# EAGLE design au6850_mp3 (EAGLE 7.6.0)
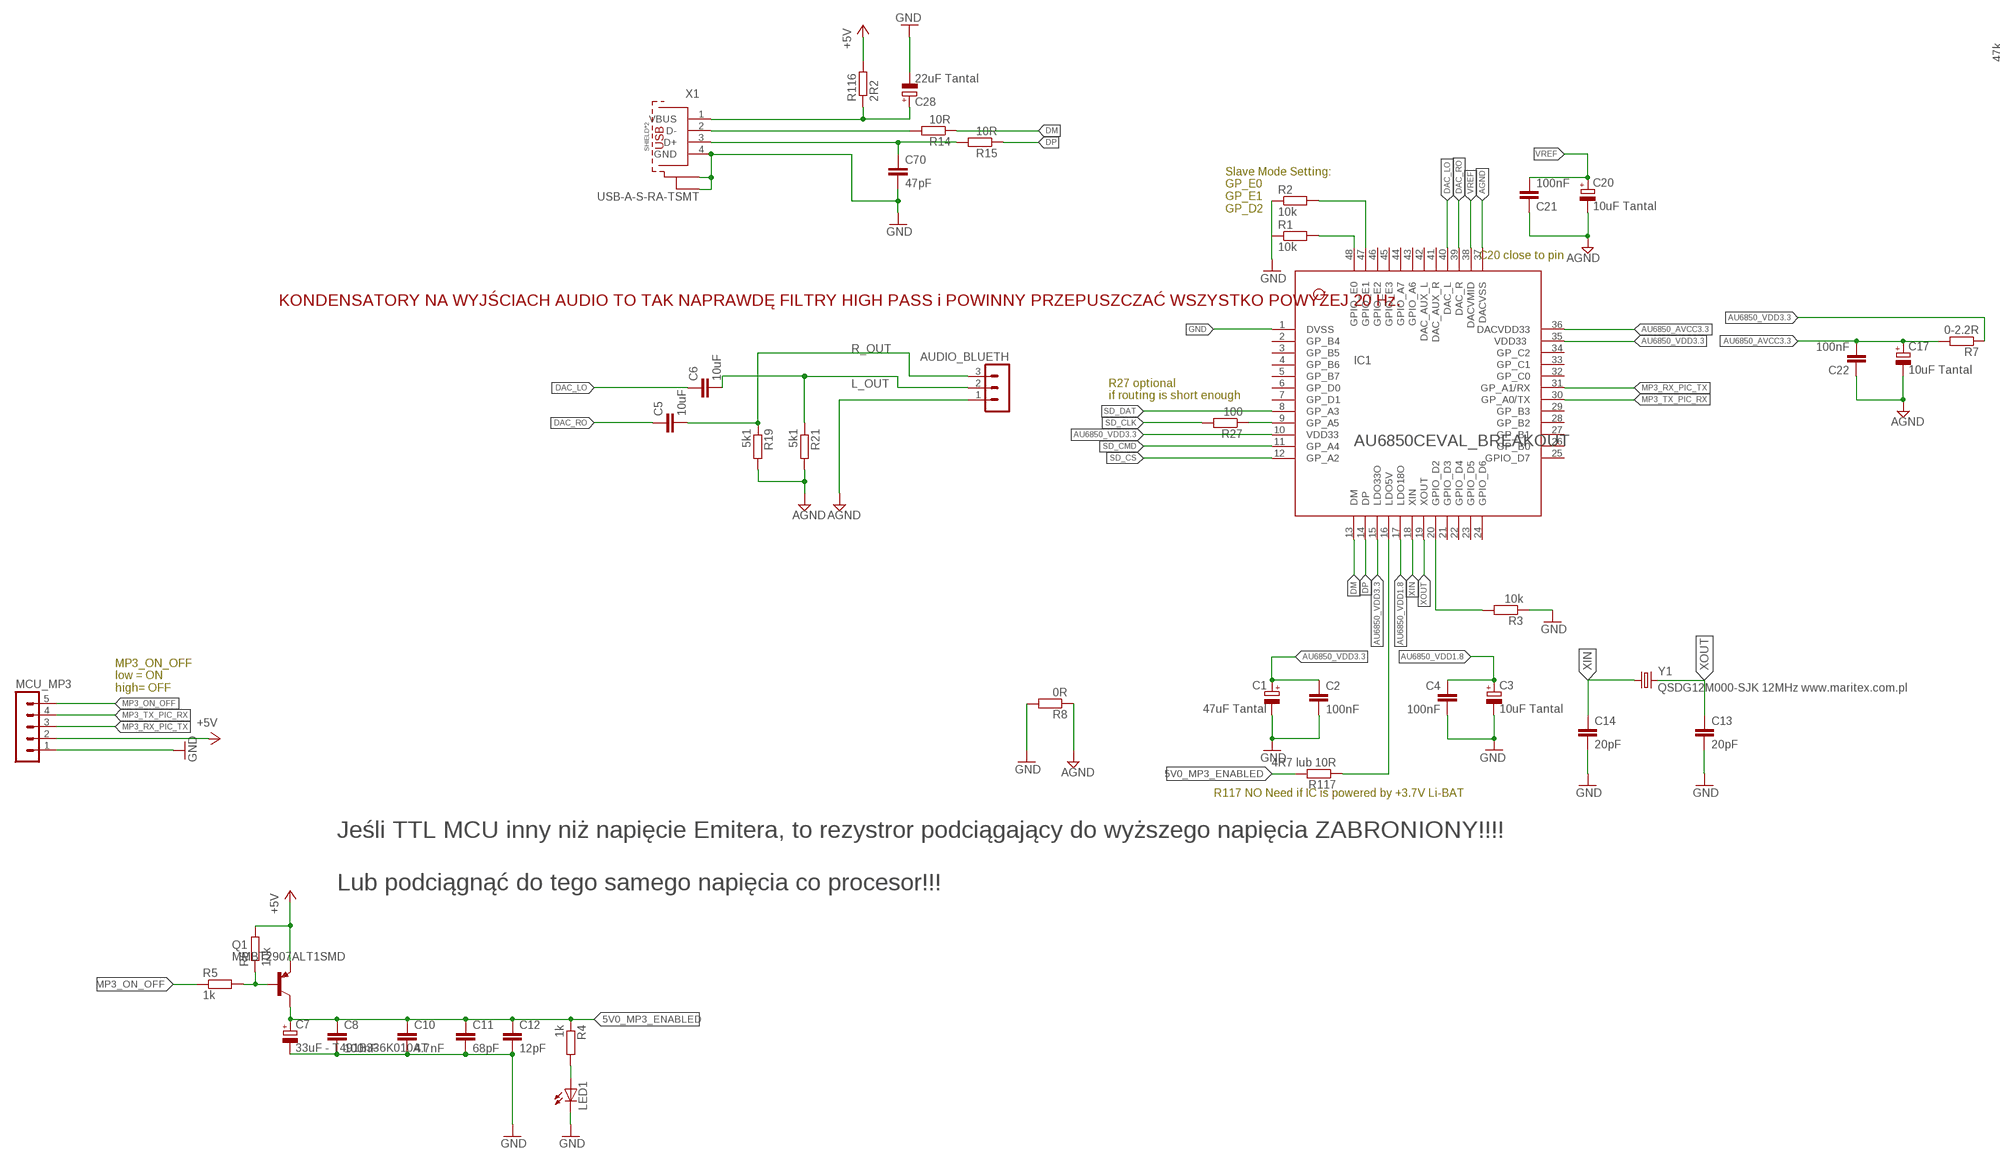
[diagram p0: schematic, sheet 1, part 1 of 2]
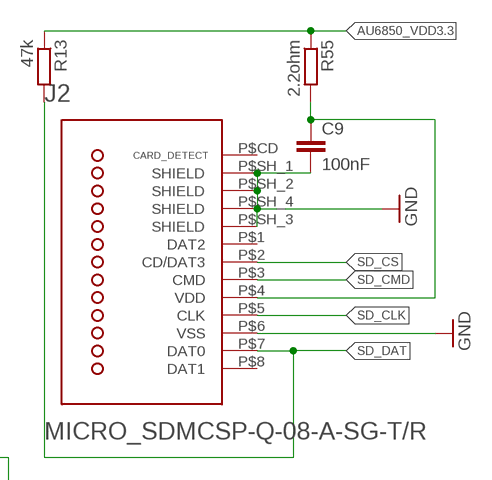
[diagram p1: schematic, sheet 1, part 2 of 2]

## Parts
AUDIO_BLUETH  MA03-1  [MA03-1]
C1  47uF Tantal  CPOL-EUB/3528-21R  [B/3528-21R]
C2  100nF  C-EUC0805  [C0805]
C3  10uF Tantal  CPOL-EUB/3528-21R  [B/3528-21R]
C4  100nF  C-EUC0805  [C0805]
C5  10uF  C-EUC0805  [C0805]
C6  10uF  C-EUC0805  [C0805]
C7  33uF - T491B336K010AT  CPOL-EUSMCB  [SMC_B]
C8  100nF  C-EUC0805  [C0805]
C9  100nF  C-EUC0805  [C0805]
C10  4.7nF  C-EUC0805  [C0805]
C11  68pF  C-EUC0805  [C0805]
C12  12pF  C-EUC0603K  [C0603K]
C13  20pF  C-EUC0805  [C0805]
C14  20pF  C-EUC0805  [C0805]
C17  10uF Tantal  CPOL-EUB/3528-21R  [B/3528-21R]
C20  10uF Tantal  CPOL-EUB/3528-21R  [B/3528-21R]
C21  100nF  C-EUC0805  [C0805]
C22  100nF  C-EUC0805  [C0805]
C28  22uF Tantal  CPOL-EUSMCB  [SMC_B]
C70  47pF  C-EUC0805  [C0805]
IC1  AU6850CEVAL_BREAKOUT  [LQFP48-7BREAKOUT]
J2  MICRO_SDMCSP-Q-08-A-SG-T/R  [MICRO_SD_8PINS]
LED1  LED3MM  [LED3MM]
MCU_MP3  MA05-1  [MA05-1]
Q1  MMBT2907ALT1SMD  [SOT23-BEC]
R1  10k  R-EU_R0805  [R0805]
R2  10k  R-EU_R0805  [R0805]
R3  10k  R-EU_R0805  [R0805]
R4  1k  R-EU_M0805  [M0805]
R5  1k  R-EU_M0805  [M0805]
R6  10k  R-EU_M0805  [M0805]
R7  0-2.2R  R-EU_R0805  [R0805]
R8  0R  R-EU_R0805  [R0805]
R13  47k  R-EU_R0805  [R0805]
R14  10R  R-EU_R0805  [R0805]
R15  10R  R-EU_R0805  [R0805]
R19  5k1  R-EU_R0805  [R0805]
R21  5k1  R-EU_R0805  [R0805]
R27  100  R-EU_R0805  [R0805]
R55  2.2ohm  R-EU_R0805  [R0805]
R116  2R2  R-EU_R0805  [R0805]
R117  4R7 lub 10R  R-EU_R0805  [R0805]
X1  USB-A-S-RA-TSMT  [USB-A-S-RA-TSMT]
Y1  QSDG12M000-SJK 12MHz www.maritex.com.pl  CRYSTALSMD  [HC49UP]

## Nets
5V0_MP3_ENABLED: C7.+ C8.1 C10.1 C11.1 C12.1 Q1.C R4.1 R117.2
+5V: MCU_MP3.2 Q1.E R6.2 R116.2
AGND: AUDIO_BLUETH.1 C17.- C20.- C21.1 C22.1 IC1.37(DACVSS) R8.1 R19.2 R21.2
AU6850_AVCC3.3: C17.+ C22.2 IC1.36(DACVDD33) R7.2
AU6850_VDD1.8: C3.+ C4.1 IC1.17(LDO18O)
AU6850_VDD3.3: C1.+ C2.1 IC1.10(VDD33) IC1.15(LDO33O) IC1.35(VDD33) R7.1 R13.1 R55.1
DAC_LO: C6.1 IC1.40(DAC_L)
DAC_RO: C5.1 IC1.39(DAC_R)
DM: IC1.13(DM) R14.1
DP: IC1.14(DP) R15.1
GND: C1.- C2.2 C3.- C4.2 C7.- C8.2 C9.2 C10.2 C11.2 C12.2 C13.2 C14.2 C28.- C70.2 IC1.1(DVSS) J2.P$6(VSS) J2.P$SH_1(1_GND_PAD) J2.P$SH_2(2_GND_PAD) J2.P$SH_3(3_GND_PAD) J2.P$SH_4(4_GND_PAD) LED1.K(C) MCU_MP3.1 R1.1 R2.1 R3.1 R8.2 X1.4(GND) X1.5(SH1) X1.6(SH2)
L_OUT: AUDIO_BLUETH.2 C6.2 R21.1
MP3_ON_OFF: MCU_MP3.5 R5.1
MP3_RX_PIC_TX: IC1.31(GP_A1/RX) MCU_MP3.3
MP3_TX_PIC_RX: IC1.30(GP_A0/TX) MCU_MP3.4
N$1: LED1.A R4.2
N$2: Q1.B R5.2 R6.1
N$4: IC1.16(LDO5V) R117.1
N$5: IC1.9(GP_A5) R27.1
N$8: C28.+ R116.1 X1.1(VBUS)
N$9: C70.1 R15.2 X1.3(D+)
N$10: R14.2 X1.2(D-)
N$14: C9.1 J2.P$4(VDD) R55.2
R_OUT: AUDIO_BLUETH.3 C5.2 R19.1
SD_CLK: J2.P$5(CLK) R27.2
SD_CMD: IC1.11(GP_A4) J2.P$3(CMD)
SD_CS: IC1.12(GP_A2) J2.P$2(CD/DAT3)
SD_DAT: IC1.8(GP_A3) J2.P$7(DAT0) R13.2
SLAVE_D2: IC1.20(GPIO_D2) R3.2
SLAVE_E0: IC1.48(GPIO_E0) R1.2
SLAVE_E1: IC1.47(GPIO_E1) R2.2
VREF: C20.+ C21.2 IC1.38(DACVMID)
XIN: C14.1 IC1.18(XIN) Y1.1
XOUT: C13.1 IC1.19(XOUT) Y1.2
Unconnected: IC1.2(GP_B4) IC1.3(GP_B5) IC1.4(GP_B6) IC1.5(GP_B7) IC1.6(GP_D0) IC1.7(GP_D1) IC1.21(GPIO_D3) IC1.22(GPIO_D4) IC1.23(GPIO_D5) IC1.24(GPIO_D6) IC1.25(GPIO_D7) IC1.26(GP_B0) IC1.27(GP_B1) IC1.28(GP_B2) IC1.29(GP_B3) IC1.32(GP_C0) IC1.33(GP_C1) IC1.34(GP_C2) IC1.41(DAC_AUX_R) IC1.42(DAC_AUX_L) IC1.43(GPIO_A6) IC1.44(GPIO_A7) IC1.45(GPIO_E3) IC1.46(GPIO_E2) J2.P$1(DAT2) J2.P$8(DAT1) J2.P$CD(CARD_DETECT_SW)

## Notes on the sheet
- Slave Mode Setting:
  GP_E0
  GP_E1
  GP_D2
- C20 close to pin
- KONDENSATORY NA WYJŚCIACH AUDIO TO TAK NAPRAWDĘ FILTRY HIGH PASS i POWINNY PRZEPUSZCZAĆ WSZYSTKO POWYŻEJ 20 Hz.
- R27 optional
  if routing is short enough
- MP3_ON_OFF
  low = ON
  high= OFF
- R117 NO Need if IC is powered by +3.7V Li-BAT
- Jeśli TTL MCU inny niż napięcie Emitera, to rezystror podciągający do wyższego napięcia ZABRONIONY!!!!
  
  Lub podciągnąć do tego samego napięcia co procesor!!!

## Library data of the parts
AUDIO_BLUETH = con-lstb:MA03-1: PIN HEADER; OC_FARNELL: unknown; OC_NEWARK: unknown
C1 = rcl:CPOL-EU: POLARIZED CAPACITOR, European symbol; PARTNUM: TAJB476K010R; SUPPLIER: TME
C2 C4-C6 C21 C22 = rcl:C-EU: CAPACITOR, European symbol
C3 = rcl:CPOL-EU: POLARIZED CAPACITOR, European symbol; PARTNUM: TAJA106K010R; SUPPLIER: TME
C7 = resistor:CPOL-EU: POLARIZED CAPACITOR, European symbol; PARTNUM: TAJB336K010R; SUPPLIER: TME
C8-C14 C70 = resistor:C-EU: CAPACITOR, European symbol
C17 C20 = rcl:CPOL-EU: POLARIZED CAPACITOR, European symbol
C28 = rcl:CPOL-EU: POLARIZED CAPACITOR, European symbol; PARTNUM: TAJB226M010R; SUPPLIER: TME
IC1 = mvsilicon:AU6850C
J2 = ADAM_TECH_SD_Card:MICRO_SD: Adam Tech; PARTNUM: MCSP-Q-08-A-SG-T/R; SUPPLIER: TME
LED1 = led:LED: LED
MCU_MP3 = con-lstb:MA05-1: PIN HEADER; OC_FARNELL: unknown; OC_NEWARK: unknown
Q1 = transistor-pnp:MMBT2907*: PNP Transistror
R1-R8 R13-R15 R19 R21 R27 R55 R116 R117 = rcl:R-EU_: RESISTOR, European symbol
X1 = ADAM_TECH_USB-A-S-RA-TSMT:USB-A-S-RA-TSMT: MULTICOMP - USB-A-S-RA-TSMT - USB, 3.0 TYPE A, RECEPTACLE, SMT CUI -UJ2-AH-1-SMT-TR, 3.0 TYPE A, RECEPTACLE, SMT AdamTech - USB-A-S-RA-TSMT - USB, 3.0 TYPE A, RECEPTACLE, SMT Source: Datasheet; DESCRIPTION: MULTICOMP - USB-A-S-RA-TSMT - USB, 3.0 TYPE A, RECEPTACLE, SMT; HEIGHT: mm; MANUFACTURER_NAME: MULTICOMP; MANUFACTURER_PART_NUMBER: USB-A-S-RA-TSMT
Y1 = SparkFun-FreqCtrl:CRYSTAL: Various standard crystals. Proven footprints. Spark Fun Electronics SKU : COM-00534; PARTNUM: 12.00M-SMDHC49S; SUPPLIER: TME

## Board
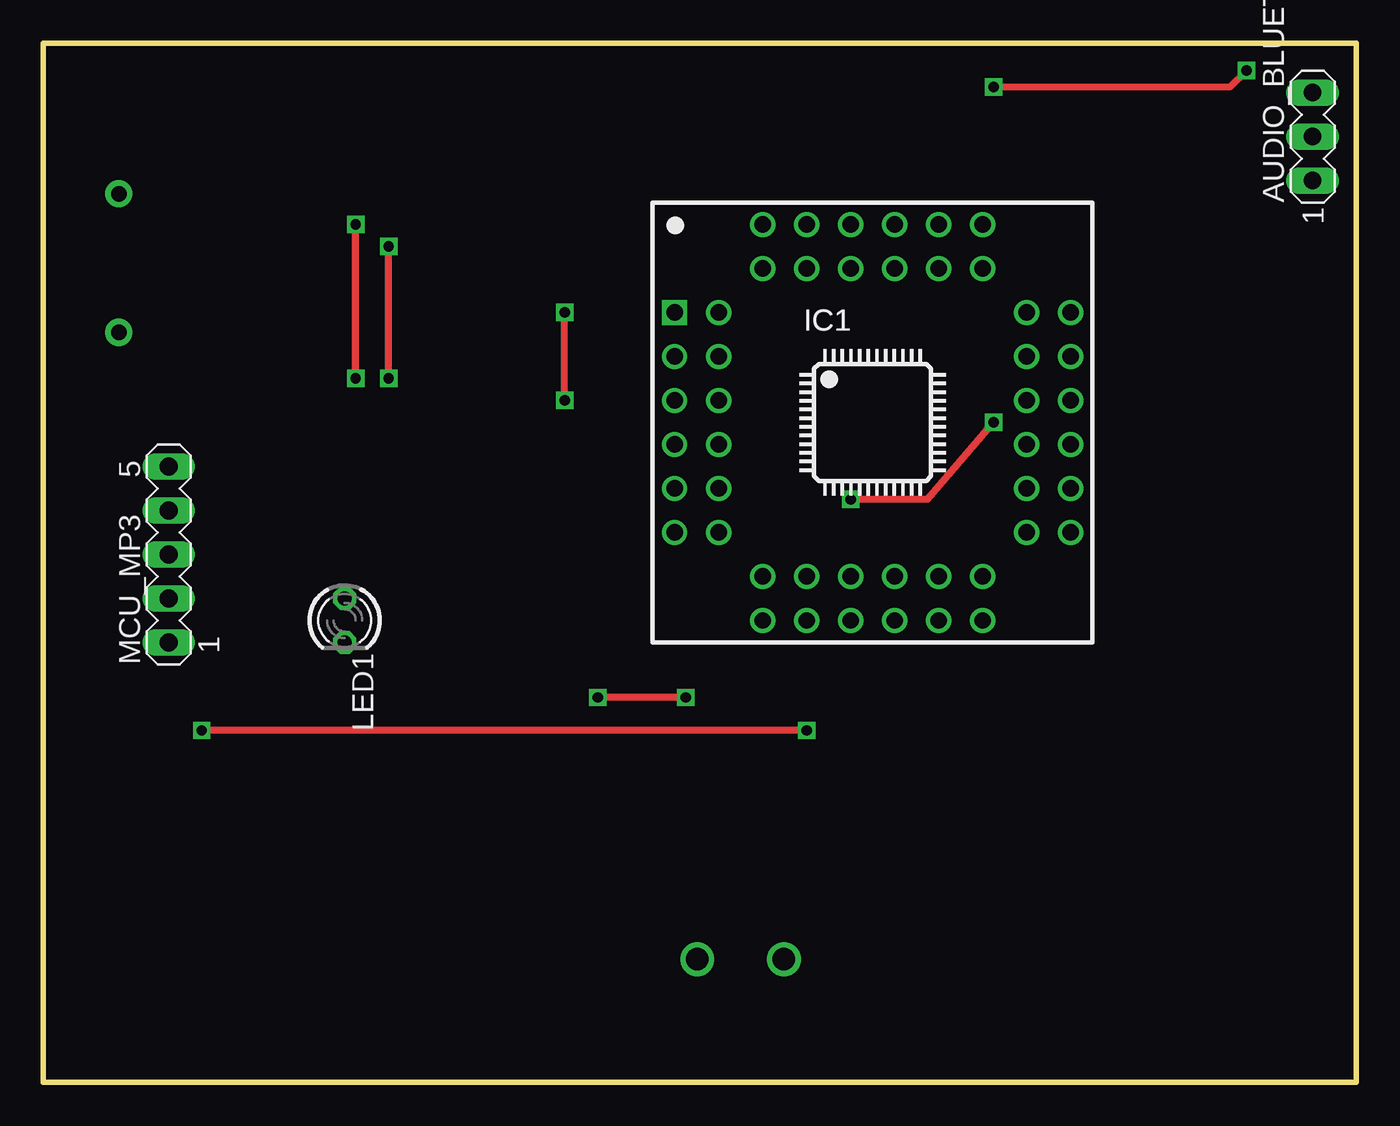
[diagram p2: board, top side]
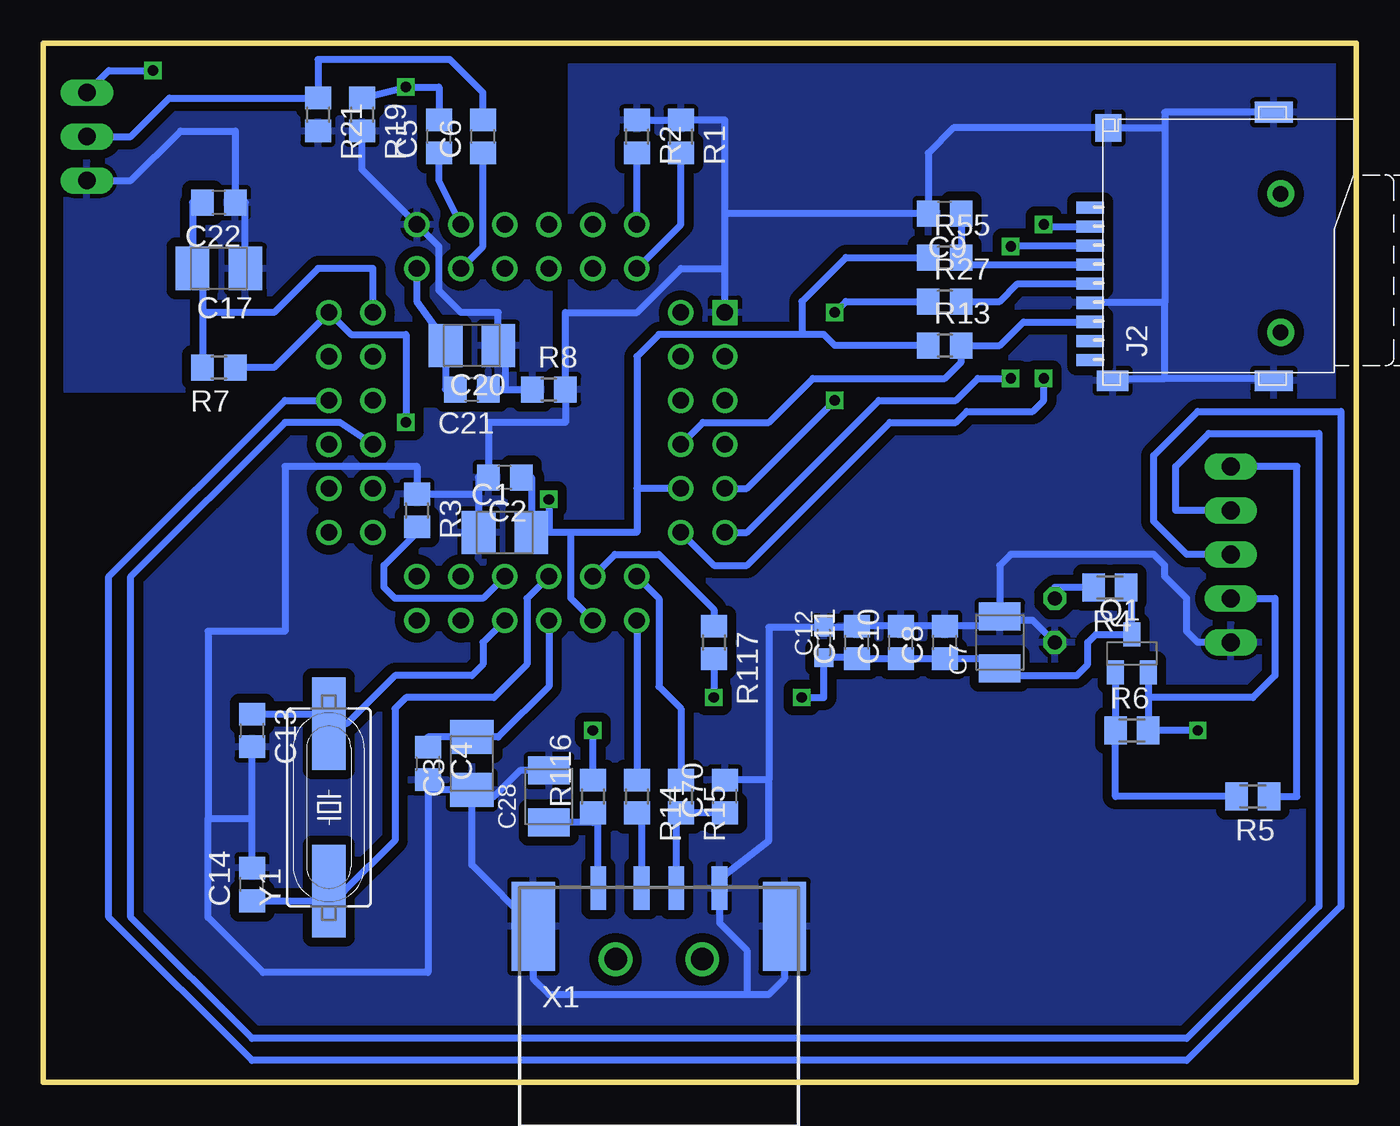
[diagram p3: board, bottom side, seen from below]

Size 75.8 x 59.99 mm. Coordinates in mm from the lower left corner, seen from the top.
Outline: 0,0 75.8,0 75.8,59.99 0,59.99 0,0
Copper layers (1*16): Top 0.035mm / dielectric 1.5mm / Bottom 0.035mm
Design rules "default": minimum track width 10mil, minimum drill 24mil, track to track 8mil, track to pad 8mil, pad to pad 8mil, via to via 8mil, smd to smd 8mil, copper to edge 40mil, drill to drill 8mil, minimum pad ring 10mil, minimum via ring 8mil, stop-mask expansion 4mil, vias tented up to drill 0mil, thermal gap 10mil

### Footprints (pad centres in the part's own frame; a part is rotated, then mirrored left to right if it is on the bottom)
MA03-1 = drill 1.016 long: 1 -2.54,0; 2 0,0; 3 2.54,0
B/3528-21R = smd 1.95 x 2.5: + 1.525,0; - -1.525,0
C0805 = smd 1.3 x 1.5: 1 -0.95,0; 2 0.95,0
SMC_B = smd 1.6 x 2.4: + -1.5,0; - 1.5,0
C0603K = smd 1.05 x 1.08: 1 -0.875,0; 2 0.875,0
LQFP48-7BREAKOUT = drill 0.95 square: 1 -11.43,6.35 | drill 0.95: 2 -8.89,6.35; 3 -11.43,3.81; 4 -8.89,3.81; 5 -11.43,1.27; 6 -8.89,1.27; 7 -11.43,-1.27; 8 -8.89,-1.27; 9 -11.43,-3.81; 10 -8.89,-3.81; 11 -11.43,-6.35; 12 -8.89,-6.35; 13 -6.35,-11.43; 14 -6.35,-8.89; 15 -3.81,-11.43; 16 -3.81,-8.89; 17 -1.27,-11.43; 18 -1.27,-8.89; 19 1.27,-11.43; 20 1.27,-8.89; 21 3.81,-11.43; 22 3.81,-8.89; 23 6.35,-11.43; 24 6.35,-8.89; 25 11.43,-6.35; 26 8.89,-6.35; 27 11.43,-3.81; 28 8.89,-3.81; 29 11.43,-1.27; 30 8.89,-1.27; 31 11.43,1.27; 32 8.89,1.27; 33 11.43,3.81; 34 8.89,3.81; 35 11.43,6.35; 36 8.89,6.35; 37 6.35,11.43; 38 6.35,8.89; 39 3.81,11.43; 40 3.81,8.89; 41 1.27,11.43; 42 1.27,8.89; 43 -1.27,11.43; 44 -1.27,8.89; 45 -3.81,11.43; 46 -3.81,8.89; 47 -6.35,11.43; 48 -6.35,8.89
MICRO_SD_8PINS = drill 0.9 pad 1.575: 1 -4.95,-10.5; 15 3.05,-10.5 | smd 0.7 x 1.6: P$1 2.25,0.5; P$2 1.15,0.5; P$3 0.05,0.5; P$4 -1.05,0.5; P$5 -2.15,0.5; P$6 -3.25,0.5; P$7 -4.35,0.5; P$8 -5.45,0.5; P$CD -6.55,0.5 | smd 1.2 x 2.2: P$SH_1 -7.75,-10.1; P$SH_2 7.75,-10.1 | smd 1.2 x 1.8: P$SH_3 -7.75,-0.8 | smd 1.6 x 1.5: P$SH_4 6.85,-0.55
LED3MM = drill 0.813 octagon: A -1.27,0; K 1.27,0
MA05-1 = drill 1.016 long: 1 -5.08,0; 2 -2.54,0; 3 0,0; 4 2.54,0; 5 5.08,0
SOT23-BEC = smd 1 x 1.4: B -0.95,-1.1; C 0,1.1; E 0.95,-1.1
R0805 = smd 1.3 x 1.5: 1 -0.95,0; 2 0.95,0
M0805 = smd 1.3 x 1.6: 1 -0.95,0; 2 0.95,0
USB-A-S-RA-TSMT = smd 0.9 x 2.5: 1 -3.5,13.75; 2 -1,13.75; 3 1,13.75; 4 3.5,13.75 | smd 2.5 x 5.15: 5 -7.25,11.55; 6 7.25,11.55 | drill 1.3 pad 1.95: 7 -2.5,9.65; 8 2.5,9.65
HC49UP = smd 5.334 x 1.93: 1 -4.826,0; 2 4.826,0

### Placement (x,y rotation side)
AUDIO_BLUETH  73.28,54.61 90 top
C1  49.15,31.75 0 bottom
C2  49.15,34.93 180 bottom
C3  51.05,18.41 90 bottom
C4  53.59,18.41 270 bottom
C5  52.96,54.61 90 bottom
C6  50.42,54.61 90 bottom
C7  20.57,25.4 90 bottom
C8  23.75,25.4 90 bottom
C9  23.75,50.16 180 bottom
C10  26.29,25.4 90 bottom
C11  28.83,25.4 90 bottom
C12  30.73,25.4 90 bottom
C13  63.75,20.32 270 bottom
C14  63.75,11.43 90 bottom
C17  65.66,46.99 180 bottom
C20  51.05,42.55 180 bottom
C21  51.05,40.01 180 bottom
C22  65.66,50.8 180 bottom
C28  46.61,16.51 90 bottom
C70  36.45,16.51 90 bottom
IC1  47.88,38.1 0 top
J2  14.86,48.26 90 bottom
LED1  17.4,26.67 270 top
MCU_MP3  7.24,30.48 90 top
Q1  12.95,24.77 0 bottom
R1  38.99,54.61 270 bottom
R2  41.53,54.61 270 bottom
R3  54.23,33.02 270 bottom
R4  14.22,28.57 180 bottom
R5  5.97,16.51 180 bottom
R6  12.95,20.32 0 bottom
R7  65.66,41.27 180 bottom
R8  46.61,40.01 0 bottom
R13  23.75,42.55 0 bottom
R14  41.53,16.51 270 bottom
R15  38.99,16.51 270 bottom
R19  57.4,55.88 270 bottom
R21  59.94,55.88 270 bottom
R27  23.75,45.09 0 bottom
R55  23.75,47.62 0 bottom
R116  44.07,16.51 90 bottom
R117  37.08,25.4 270 bottom
X1  40.26,-2.54 0 bottom
Y1  59.31,15.88 90 bottom

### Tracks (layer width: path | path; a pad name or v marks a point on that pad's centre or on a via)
5V0_MP3_ENABLED  (via drill 0.6)
  Top 0.406: v37.08,22.23 v32,22.23
  Bottom 0.406: R4.1 arc90 12.95,28.26 Q1.C 15.03,25.87 15.49,25.4 15.49,24.13 16.13,23.5 20.17,23.5 C7.+ 21.12,24.45 C8.1 C10.1 C11.1 28.9,24.53 C12.1 30.73,22.23 v32,22.23 | R117.2 v37.08,22.23
+5V  (via drill 0.6)
  Top 0.406: v44.07,20.32 v9.14,20.32
  Bottom 0.406: Q1.E 12,22.23 | 12,22.23 R6.2 v9.14,20.32 | MCU_MP3.2 4.7,27.94 4.7,23.5 5.97,22.23 12,22.23 | R116.2 v44.07,20.32
AGND
  Bottom 0.406: AUDIO_BLUETH.1 70.74,52.07 67.88,54.93 64.71,54.93 C22.1 | C22.1 64.39,50.8 | C17.- 64.13,50.8 C22.1 | C21.1 49.15,40.01 | 49.15,40.01 R8.1 | 49.15,40.01 49.15,42.16 C20.- 49.53,44.45 51.69,44.45 52.96,45.72 52.96,48.26 IC1.37 57.4,52.7 R19.2
  pour Bottom (isolate 0.533): 46.61,40.01 79.63,40.01 79.63,62.23 46.61,62.23
AU6850_AVCC3.3
  Bottom 0.406: C22.2 67.18,50.8 C17.+ 66.61,46.99 66.61,44.45 | 66.61,44.45 R7.2 | IC1.36 56.77,46.99 59.94,46.99 62.48,44.45 66.61,44.45
AU6850_VDD1.8
  Bottom 0.406: IC1.17 46.61,22.86 49.53,19.94 C3.+ 53.59,19.94 C4.1
AU6850_VDD3.3  (via drill 0.6)
  Top 0.406: v54.86,38.1 51.05,33.66 v46.61,33.66
  Bottom 0.406: IC1.15 45.34,27.94 45.34,31.75 | IC1.10 41.53,34.29 | R7.1 62.48,41.27 IC1.35 58.04,43.18 54.86,43.18 v54.86,38.1 | R13.1 30.1,42.55 30.73,43.18 32,43.18 | 32,43.18 40.26,43.18 41.53,41.91 41.53,34.29 | 32,43.18 32,45.09 29.46,47.62 R55.1 | 41.53,34.29 41.53,31.75 45.34,31.75 | 45.34,31.75 46.61,31.75 | 46.61,31.75 C1.+ 47.62,34.93 C2.1 | v46.61,33.66 46.61,31.75
DAC_LO
  Bottom 0.406: IC1.40 50.42,48.26 C6.1
DAC_RO
  Bottom 0.406: IC1.39 52.96,52.07 C5.1
DM
  Bottom 0.406: IC1.13 R14.1
DP
  Bottom 0.406: IC1.14 40.26,27.94 40.26,22.86 38.99,21.59 R15.1
GND
  Bottom 0.406: R2.1 R1.1 36.45,55.56 36.45,50.16 | C28.- 48.28,18.01 49.78,16.51 50.67,16.51 C3.- | 35.18,5.08 46.61,5.08 47.51,5.98 X1.5 51.05,12.55 C3.- | 35.18,5.08 33.91,5.08 33.01,5.98 X1.6 | 35.18,5.08 35.18,7.62 36.76,9.2 X1.4 36.76,11.75 33.91,13.97 33.91,17.46 | C3.- 53.59,16.89 | 53.59,16.89 C4.2 | 53.59,16.89 53.59,6.35 63.12,6.35 66.29,9.52 66.29,15.24 | 33.91,17.46 C70.2 | IC1.1 36.45,46.99 | 36.45,46.99 36.45,50.16 | 36.45,46.99 38.99,46.99 41.53,44.45 45.66,44.45 R8.2 45.66,38.1 50.1,38.1 C2.2 50.67,34.93 C1.- 50.67,33.97 R3.1 | C7.- 21.12,26.35 C8.2 C10.2 C11.2 28.9,26.28 C12.2 33.91,26.28 33.91,17.46 | LED1.K 18.67,26.67 19.94,26.67 20.17,26.9 C7.- | 36.45,50.16 C9.2 24.7,53.66 23.25,55.11 J2.P$SH_4 11.05,55.11 | J2.P$SH_3 13.93,40.64 11.05,40.64 | 11.05,40.64 11.05,45.01 | 11.05,45.01 J2.P$6 | J2.P$SH_1 4.76,40.64 11.05,40.64 | J2.P$SH_2 11.05,56.01 11.05,55.11 | 11.05,55.11 11.05,45.01 | C14.2 63.75,15.24 | 63.75,15.24 C13.2 | 66.29,15.24 63.75,15.24 | R3.1 54.54,33.97 | 66.29,15.24 66.29,26.04 61.85,26.04 61.85,35.56 54.23,35.56 R3.1 | MCU_MP3.1 9.14,25.4 9.78,26.04 9.78,27.94 11.05,29.21 11.05,29.84 11.68,30.48 19.94,30.48 20.57,29.84 C7.-
  pour Bottom (isolate 0.533): -1.65,-2.54 -2.92,-2.54 -2.92,62.23 45.34,62.23 45.34,38.73 79.63,38.73 79.63,-6.35 -1.65,-6.35
L_OUT
  Bottom 0.406: AUDIO_BLUETH.2 70.74,54.61 68.52,56.83 R21.1 59.94,59.05 52.32,59.05 50.42,57.15 C6.2
MP3_ON_OFF
  Bottom 0.406: R5.1 3.43,16.51 3.43,35.56 MCU_MP3.5
MP3_RX_PIC_TX
  Bottom 0.406: MCU_MP3.3 9.78,30.48 11.68,32.38 11.68,36.2 9.14,38.73 0.89,38.73 0.89,10.16 9.78,1.27 63.75,1.27 72.01,9.52 72.01,29.21 61.85,39.37 IC1.31
MP3_TX_PIC_RX
  Bottom 0.406: MCU_MP3.4 10.41,33.02 10.41,35.56 8.51,37.47 2.16,37.47 2.16,10.16 9.78,2.54 63.75,2.54 70.74,9.52 70.74,29.21 61.85,38.1 58.67,38.1 IC1.30
N$1
  Bottom 0.406: R4.2 17.4,28.57 LED1.A
N$2
  Bottom 0.406: R5.2 13.9,16.51 R6.1 Q1.B
N$4
  Bottom 0.406: IC1.16 42.8,30.48 40.26,30.48 37.08,27.3 R117.1
N$5  (via drill 0.6)
  Top 0.406: v30.1,39.37 v30.1,44.45
  Bottom 0.406: IC1.9 35.18,34.29 v30.1,39.37 | v30.1,44.45 29.46,45.09 R27.1
N$8
  Bottom 0.406: C28.+ 44.07,15.01 R116.1 43.76,15.56 X1.1
N$9
  Bottom 0.406: X1.3 39.26,15.29 arc90 R15.2 C70.1
N$10
  Bottom 0.406: R14.2 arc90 41.26,15.29 X1.2
N$14
  Bottom 0.406: C9.1 R55.2 22.8,47.21 J2.P$4
R_OUT  (via drill 0.6)
  Top 0.406: v69.47,58.42 68.51,57.47 v54.86,57.47
  Bottom 0.406: AUDIO_BLUETH.3 72.01,58.42 v69.47,58.42 | C5.2 52.96,57.47 v54.86,57.47 R19.1
SD_CLK
  Bottom 0.406: R27.2 20.57,45.09 19.55,46.11 J2.P$5
SD_CMD  (via drill 0.6)
  Top 0.406: v19.94,40.64 v19.94,48.26
  Bottom 0.406: IC1.11 35.18,31.75 27.56,39.37 23.11,39.37 21.84,40.64 v19.94,40.64 | v19.94,48.26 19.89,48.31 J2.P$3
SD_CS  (via drill 0.6)
  Top 0.406: v18.03,40.64 v18.03,49.53
  Bottom 0.406: IC1.12 37.08,29.84 35.18,29.84 26.92,38.1 23.11,38.1 22.48,38.73 18.67,38.73 18.03,39.37 v18.03,40.64 | v18.03,49.53 17.91,49.41 J2.P$2
SD_DAT
  Bottom 0.406: J2.P$7 19.21,43.91 20.57,42.55 R13.2 22.8,41.59 23.75,40.64 31.37,40.64 33.91,38.1 37.72,38.1 IC1.8
SLAVE_D2
  Bottom 0.406: IC1.20 50.42,27.94 55.5,27.94 56.13,28.57 56.13,29.84 54.23,31.75 R3.2
SLAVE_E0
  Bottom 0.406: IC1.48 38.99,49.53 R1.2
SLAVE_E1
  Bottom 0.406: IC1.47 R2.2
VREF
  Bottom 0.406: IC1.38 54.23,45.09 52.58,42.8 C20.+ 52.58,40.01 C21.2
XIN
  Bottom 0.406: IC1.18 47.88,27.94 47.88,24.13 49.78,22.23 54.86,22.23 55.5,21.59 55.5,13.97 58.42,11.05 Y1.1 59.31,10.48 C14.1
XOUT
  Bottom 0.406: IC1.19 50.42,25.4 50.42,24.13 51.05,23.5 55.5,23.5 58.29,20.7 Y1.2 59.31,21.27 C13.1

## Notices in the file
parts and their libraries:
SparkFun-FreqCtrl: Licensing: Creative Commons ShareAlike 4.0 International - https://creativecommons.org/licenses/by-sa/4.0
